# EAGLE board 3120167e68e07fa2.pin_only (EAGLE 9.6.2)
REV: B

Size 11.43 x 17.78 mm. Coordinates in mm from the lower left corner, seen from the top.
Outline: 0,0 0,15.24 arc-90 2.54,17.78 8.89,17.78 arc-90 11.43,15.24 11.43,0 0,0
Copper layers (1*16): Top 0.035mm / dielectric 1.5mm / Bottom 0.035mm
Design rules "adafruit 7-7": minimum track width 6mil, minimum drill 15.5mil, track to track 8mil, track to pad 7mil, pad to pad 7mil, via to via 7mil, smd to smd 7mil, copper to edge 10mil, drill to drill 8mil, minimum pad ring 10mil, minimum via ring 8mil, stop-mask expansion 2mil, vias tented up to drill 20mil, thermal gap 10mil

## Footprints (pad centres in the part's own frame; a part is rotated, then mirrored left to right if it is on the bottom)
0805-NO = smd 1.24 x 1.5: 1 -0.95,0; 2 0.95,0
FIDUCIAL_1MM = smd 1 x 1: 1 0,0
SOT563 = smd 0.65 x 0.275: 1 -0.635,0.5; 2 -0.635,0; 3 -0.635,-0.5; 4 0.635,-0.5; 5 0.635,0; 6 0.635,0.5
1X04_ROUND = drill 1 pad 1.778: 1 -3.81,0; 2 -1.27,0; 3 1.27,0; 4 3.81,0
INDUCTOR_5X5MM_TDK_VLC5045 = smd 2 x 5: P$1 -1.6,0; P$2 1.6,0
0603-NO = smd 1.075 x 1: 1 -0.85,0; 2 0.85,0
MOUNTINGHOLE_2.5_PLATED = drill 2.5 pad 3.2: P$1 0,0

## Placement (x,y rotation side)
C1  22uF  [0805-NO]  8.26,6.6 180 top
C2  22uF  [0805-NO]  3.17,4.7 0 top
C3  22uF  [0805-NO]  8.26,4.72 180 top
FID1  FIDUCIAL_1MM  [FIDUCIAL_1MM]  9.53,16.13 0 top
IC1  TPS61023  [SOT563]  7.87,8.76 270 top
JP1  [1X04_ROUND]  5.71,2.54 180 top
L1  1uH  [INDUCTOR_5X5MM_TDK_VLC5045]  3.68,8.76 270 top
R1  100K  [0603-NO]  8.13,11.56 270 top
R2  732K  [0603-NO]  9.65,8.99 90 top
R3  100K  [0603-NO]  9.65,12.06 90 top
U$9  MOUNTINGHOLE2.5  [MOUNTINGHOLE_2.5_PLATED]  2.54,15.24 0 top
U$10  [PCBFEAT-REV-040]  6.22,14.86 0 bottom
U$11  [ADAFRUIT_2.5MM]  10.03,14.22 0 bottom

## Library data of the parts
C1-C3 JP1 L1 R1-R3 U$11 = microbuilder
FID1 U$9 = microbuilder; BOM: EXCLUDE
IC1 = adafruit_power
U$10 = microbuilder; REV: B

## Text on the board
tPlace: TPS / 61023 | Vin | GND | 5V | En
bPlace: Vin: 2-5V / Vout:5V / 1A Max | TPS61023 | Vin | GND | 5V | En

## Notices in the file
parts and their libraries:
microbuilder: This work is placed in the public domain, and may be freely used for commercial and non-commercial work with the following conditions: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
